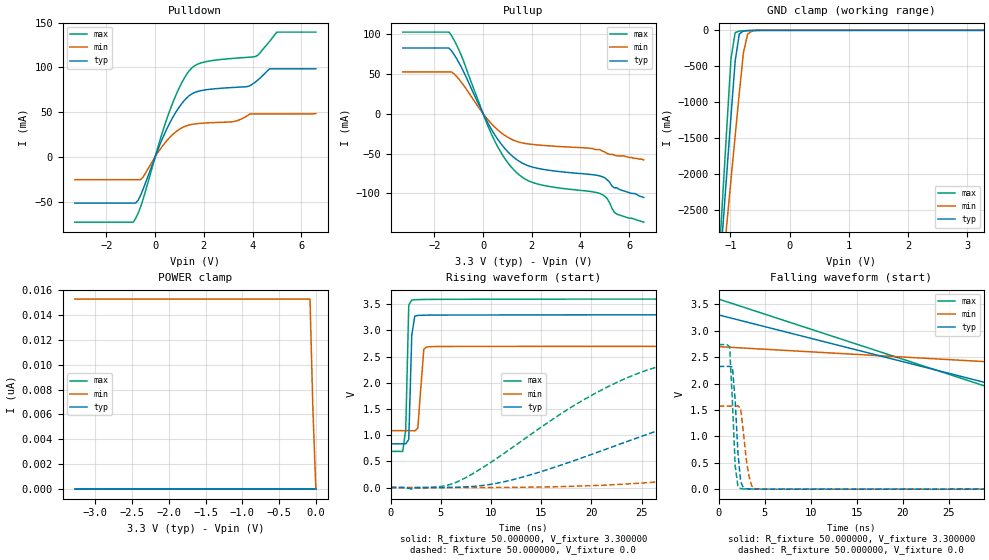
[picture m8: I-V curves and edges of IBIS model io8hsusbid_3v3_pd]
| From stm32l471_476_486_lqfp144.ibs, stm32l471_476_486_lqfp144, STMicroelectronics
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|   Model io8hsusbid_3v3_pd
[Model]  io8hsusbid_3v3_pd
Model_type I/O
Polarity   Non-Inverting
Enable   Active-Low
Vinl =   0.990000V
Vinh =   2.310000V
Vmeas =  1.650000V
Cref =   100.000000nF
Rref =   1.000000k
Vref =   3.300000V
C_comp   2.116400pF   2.092700pF   2.152900pF
[Temperature Range]   25.000000   0.125000k   -40.000000
[Pullup Reference]   3.300000V   2.700000V   3.600000V
[Pulldown Reference]   0.0V   0.0V   0.0V
[POWER Clamp Reference]   3.300000V   2.700000V   3.600000V
[GND Clamp Reference]   0.0V   0.0V   0.0V
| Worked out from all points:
|   slope of the pulldown table from 0 to 0.495 V, typ, clamps not added: 15.4 ohm
|   slope of the pullup table from 0 to 0.495 V, typ, clamps not added: 18.1 ohm
|   GND clamp passes 1 mA (typ) near -0.59 V on its own axis
|   rising waveform, R_fixture 50.000000, V_fixture 3.300000: 20-80 % time 223ps typ, 384ps min, 221ps max; typ from 0.835 V to 3.3 V
|   rising waveform, R_fixture 50.000000, V_fixture 0.0: 20-80 % time 23.9ns typ, 50.4ns min, 14.3ns max; typ from 0 V to 2.32 V
|   falling waveform, R_fixture 50.000000, V_fixture 3.300000: 20-80 % time 33.5ns typ, 61.1ns min, 30.7ns max; typ from 3.3 V to 0.835 V
|   falling waveform, R_fixture 50.000000, V_fixture 0.0: 20-80 % time 509ps typ, 661ps min, 429ps max; typ from 2.32 V to 0 V
[Pulldown]
|Voltage   I(typ)   I(min)   I(max)
-3.3V     -51.63mA   -25.53mA   -73.04mA
-900mV    -51.63mA   -25.53mA   -73.04mA
-500mV    -36.51mA   -22.8mA    -47.71mA
200mV     14.02mA    8.316mA    18.9mA
700mV     42.99mA    24.4mA     58.9mA
1.2V      63.06mA    33.8mA     88.14mA
1.6V      71.63mA    36.67mA    101.4mA
3.2V      77.51mA    39.29mA    110mA
4.1V      83.27mA    48mA       111.9mA
4.7V      98.3mA     48mA       129mA
5V        98.3mA     48mA       139.4mA
6.6V      98.3mA     48.43mA    139.4mA
[Pullup]
|Voltage   I(typ)   I(min)   I(max)
-3.3V     82.22mA    52.22mA    102.1mA
-1.4V     82.22mA    52.22mA    102.1mA
-900mV    58.55mA    39.64mA    73.33mA
100mV     -6.166mA   -3.962mA   -8.038mA
500mV     -27.53mA   -17.49mA   -35.6mA
1V        -47.29mA   -29.37mA   -60.81mA
1.5V      -60.05mA   -35.95mA   -77.15mA
2.4V      -69.45mA   -39.66mA   -89.34mA
4.8V      -78.1mA    -45mA      -100.1mA
5.1V      -83mA      -50mA      -106.7mA
5.5V      -93mA      -53mA      -126mA
6.6V      -105mA     -58mA      -136mA
[GND_clamp]
|Voltage   I(typ)   I(min)   I(max)
-3.3V     -9.914A    -9.595A    -9.188A
-1.2V     -3.541A    -3.911A    -3.279A
-1.13V    -2.75A     -3.295A    -2.301A
-1.06V    -1.963A    -2.68A     -1.33A
-990mV    -1.183A    -2.069A    -386.7mA
-920mV    -424.7mA   -1.463A    -31.42mA
-850mV    -49.13mA   -868.7mA   -10.49mA
-780mV    -9.132mA   -308.3mA   -6.726mA
-710mV    -3.661mA   -53.82mA   -3.996mA
-640mV    -1.738mA   -11.05mA   -1.896mA
-430mV    -33.31uA   -129.6uA   -18.85uA
3.28V     86.93uA    88.78uA    71.45uA
[POWER_clamp]
|Voltage   I(typ)   I(min)   I(max)
-3.28V    0A         15.27nA    0A
-80mV     0A         15.27nA    0A
-40mV     0A         6.354nA    0A
0V        0A         0A         0A
[Ramp]
| variable   typ   min   max
dV/dt_r  1.39404/23.91093n   0.94416/53.26977n   1.64262/14.30157n
dV/dt_f  1.47860/21.09034n   0.96750/44.71088n   1.74566/13.58933n
R_load = 50.000000
[Rising Waveform]
R_fixture= 50.000000
V_fixture= 3.300000
V_fixture_min= 2.700000
V_fixture_max= 3.600000
|time   V(typ)   V(min)   V(max)
0s        834.7mV    1.086V     689.8mV
1.201ns   834.6mV    1.086V     687.9mV
1.502ns   833.5mV    1.086V     1.115V
1.802ns   918.5mV    1.086V     3.487V
2.102ns   2.91V      1.085V     3.581V
2.402ns   3.273V     1.082V     3.587V
2.703ns   3.286V     1.132V     3.589V
3.303ns   3.291V     2.644V     3.591V
3.904ns   3.293V     2.69V      3.593V
149.5ns   3.299V     2.699V     3.599V
[Rising Waveform]
R_fixture= 50.000000
V_fixture= 0.0
V_fixture_min= 0.0
V_fixture_max= 0.0
|time   V(typ)   V(min)   V(max)
0s        3.142nV    58.62nV    2.998nV
6.306ns   2.707mV    -142.9uV   82.36mV
12.01ns   141.4mV    1.948mV    748.3mV
18.32ns   516.4mV    25.35mV    1.572V
23.72ns   889.5mV    70.25mV    2.109V
33.93ns   1.521V     231.2mV    2.549V
45.95ns   1.997V     483mV      2.667V
65.47ns   2.229V     894.3mV    2.722V
99.4ns    2.308V     1.373V     2.736V
149.5ns   2.323V     1.574V     2.738V
[Falling Waveform]
R_fixture= 50.000000
V_fixture= 3.300000
V_fixture_min= 2.700000
V_fixture_max= 3.600000
|time   V(typ)   V(min)   V(max)
0s        3.299V     2.699V     3.599V
50.05ns   1.088V     2.207V     752.5mV
100.1ns   862.5mV    1.296V     694.5mV
150.2ns   839.9mV    1.146V     690.2mV
200.2ns   835.7mV    1.105V     689.8mV
300.3ns   834.7mV    1.089V     689.8mV
4.955us   834.7mV    1.086V     689.8mV
[Falling Waveform]
R_fixture= 50.000000
V_fixture= 0.0
V_fixture_min= 0.0
V_fixture_max= 0.0
|time   V(typ)   V(min)   V(max)
0s        2.323V     1.574V     2.738V
1.201ns   2.323V     1.574V     2.69V
1.502ns   2.317V     1.574V     1.656V
1.802ns   1.675V     1.573V     440.5mV
2.102ns   687.8mV    1.579V     50.73mV
2.402ns   141.9mV    1.524V     10.48mV
2.703ns   21.6mV     1.06V      4.6mV
3.604ns   2.445mV    62.01mV    1.837mV
4.505ns   1.304mV    2.469mV    1.168mV
149.5ns   3.142nV    58.62nV    2.998nV
